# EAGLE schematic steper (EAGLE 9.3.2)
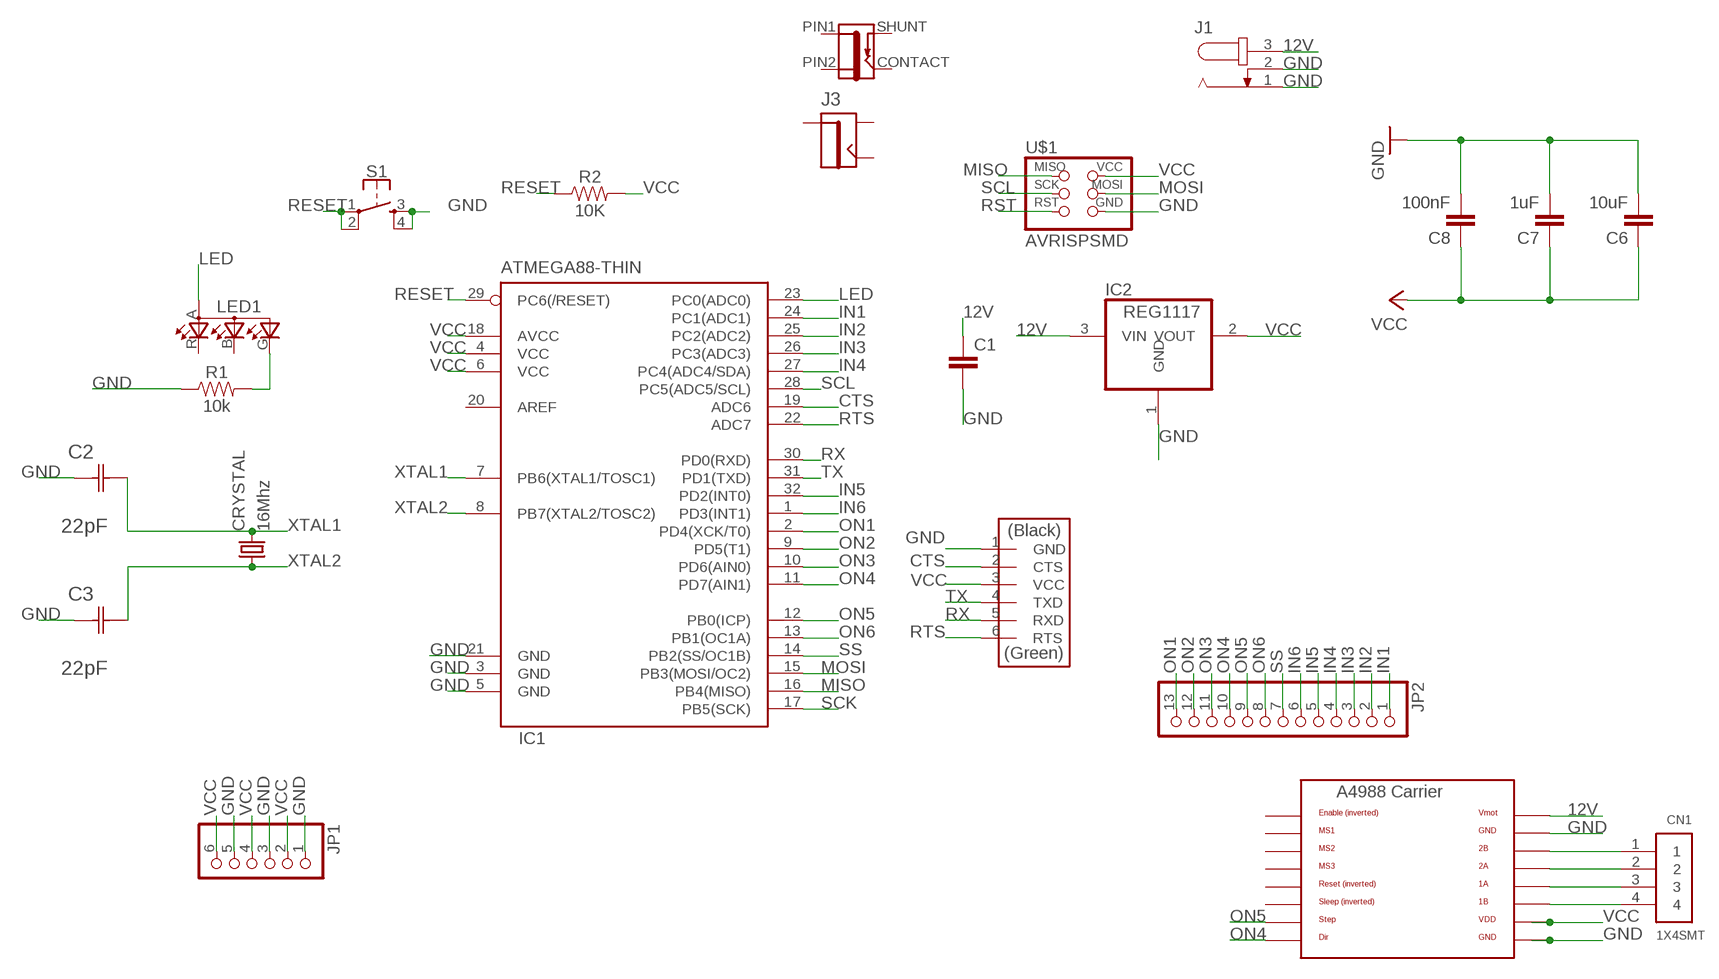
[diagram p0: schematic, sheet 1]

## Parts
C1  C2.5/2  [C2.5-2]
C2  22pF  0612ZC225MAT2A  [CAPC3216X178N]
C3  22pF  0612ZC225MAT2A  [CAPC3216X178N]
C6  10uF  CAP1206  [1206]
C7  1uF  CAP1206  [1206]
C8  100nF  CAP1206  [1206]
CN1  1X4SMT  [1X4-SMT]
CRYSTAL  16Mhz  CSM-7X-DU  [CSM-7X-DU]
IC1  ATMEGA88-THIN  [TQFP32-08THIN]
IC2  REG1117  [SOT223]
J1  JACK-PLUG1  [SPC4078]
J2  JACK-2.1MM  [PJ-002AH-SMT]
J3  JACK2.1MM  [JACK_2.1MM]
JP1  PINHD-1X61X06_SMT  [1X06_SMT]
JP2  PINHD-1X131X13_SMT  [1X13_SMT]
LED1  LEDRGBOLD  [P-LCC-4-3]
R1  10k  10KOHM-0603-1/10W-1%  [0603]
R2  10K  1OHM-0603-1/10W-1%  [0603]
S1  MOMENTARY-SWITCH-SPST-2-SMD-4.6X2.8MM  [TACTILE_SWITCH_SMD_4.6X2.8MM]
U$1  AVRISPSMD  [2X03SMD]
U$2  FTDI-SMD-HEADER  [1X06SMD]
U$4  A4988BREAKOUT  [A4988BREAKOUT]

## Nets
12V: C1.1 IC2.3(VIN) J1.3 U$4.VMOT
CTS: IC1.19(ADC6) U$2.2(CTS)
GND: C1.2 C2.1(C1) C3.1(C1) C6.2 C7.2 C8.2 IC1.3(GND) IC1.5(GND) IC1.21(GND) IC2.1(GND) J1.1 J1.2 JP1.1 JP1.3 JP1.5 R1.1 S1.3 S1.4 U$1.6(GND) U$2.1(GND) U$4.GND U$4.GND@0(GND)
IN1: IC1.24(PC1(ADC1)) JP2.1
IN2: IC1.25(PC2(ADC2)) JP2.2
IN3: IC1.26(PC3(ADC3)) JP2.3
IN4: IC1.27(PC4(ADC4/SDA)) JP2.4
IN5: IC1.32(PD2(INT0)) JP2.5
IN6: IC1.1(PD3(INT1)) JP2.6
LED: IC1.23(PC0(ADC0)) LED1.A(A2)
MISO: IC1.16(PB4(MISO)) U$1.1(MISO)
MOSI: IC1.15(PB3(MOSI/OC2)) U$1.4(MOSI)
N$1: U$4.STEP
N$2: U$4.DIR
N$3: CN1.1 U$4.2B
N$4: CN1.2 U$4.2A
N$5: CN1.3 U$4.1A
N$6: CN1.4 U$4.1B
N$18: LED1.G(CGREEN) R1.2
ON1: IC1.2(PD4(XCK/T0)) JP2.13
ON2: IC1.9(PD5(T1)) JP2.12
ON3: IC1.10(PD6(AIN0)) JP2.11
ON4: IC1.11(PD7(AIN1)) JP2.10
ON5: IC1.12(PB0(ICP)) JP2.9
ON6: IC1.13(PB1(OC1A)) JP2.8
RESET: IC1.29(PC6(/RESET)) R2.1 S1.1 S1.2
RST: U$1.5(RST)
RTS: IC1.22(ADC7) U$2.6(RTS)
RX: IC1.30(PD0(RXD)) U$2.5(RXD)
SCK: IC1.17(PB5(SCK))
SCL: IC1.28(PC5(ADC5/SCL)) U$1.3(SCK)
SS: IC1.14(PB2(SS/OC1B)) JP2.7
TX: IC1.31(PD1(TXD)) U$2.4(TXD)
VCC: C6.1 C7.1 C8.1 IC1.4(VCC) IC1.6(VCC) IC1.18(AVCC) IC2.2(VOUT) JP1.2 JP1.4 JP1.6 R2.2 U$1.2(VCC) U$2.3(VCC) U$4.VDD
XTAL1: C2.2(C2) CRYSTAL.2 IC1.7(PB6(XTAL1/TOSC1))
XTAL2: C3.2(C2) CRYSTAL.1 IC1.8(PB7(XTAL2/TOSC2))
Unconnected: IC1.20(AREF) J3.CONTACT J3.PIN J3.SHUNT LED1.B(CBLUE) LED1.R(CRED) U$4.EN U$4.MS1 U$4.MS2 U$4.MS3 U$4.RST U$4.SLP(SLEEP)

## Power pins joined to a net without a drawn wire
CONTACT: J2.CONTACT
PIN1: J2.PIN1
PIN2: J2.PIN2
SHUNT: J2.SHUNT

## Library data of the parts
C1 = capacitor-wima:C: CAPACITOR
C2 C3 = AVX_By_element14_Batch_1:0612ZC225MAT2A: Capacitor 1206; MPN: 0612ZC225MAT2A; OC_FARNELL: -; OC_NEWARK: 12N3209; SUPPLIER: AVX; TOLERANCE: ±20%; VALUE: 2.2µF; VOLTAGERATING: 10V
C6-C8 = 01_SparkFun:CAP: Capacitor
CN1 = adafruit:1X4: 4-pin connector
CRYSTAL = 01_FAB_Hello:CSM-7X-DU: SMD CRYSTAL; OC_FARNELL: unknown; OC_NEWARK: unknown
IC1 = fab:ATMEGA88-THIN
IC2 = burr-brown:REG1117: 800mA and 1A Low Dropout (LDO) Positive Regulator 1.8V, 2.5V, 2.85V, 3.3V, 5V, and Adj; MPN: REG1117; OC_FARNELL: 1097566; OC_NEWARK: 14P6981
J1 = con-jack:JACK-PLUG: DC POWER JACK Power Jack, DC, Right Angle, Through Hole, Rated 5A at 16VDC, PC Terminals Distributor: Farnell (www.Farnell.de) Drawing: 84N1161.pdf / 84N1162.pdf Manufacturer: SPC Technology (www.spctechnology.com) Type: SPC4077 / SPC 4078; OC_FARNELL: unknown; OC_NEWARK: unknown
J2 = fab:JACK-2.1MM: SMD DC power jack PJ-002AH-SMT As found in the fablab inventory. Made by Zaerc.
J3 = fab:JACK
JP1 = smd_con:PINHD-1X6: PIN HEADER
JP2 = smd_con:PINHD-1X13: PIN HEADER
LED1 = fab:LEDRGBOLD: OSRAM Hyper Multi TOPLED® Hyper-Bright LED LATB T686 Source: http://www.osram.convergy.de/
R1 = SparkFun-Resistors:10KOHM: 10kΩ resistor; PROD_ID: RES-00824
R2 = SparkFun-Resistors:1OHM: 1Ω resistor; PROD_ID: RES-08269; VALUE: 1
S1 = SparkFun-Switches:MOMENTARY-SWITCH-SPST-2: Momentary Switch (Pushbutton) - SPST - Two Circuits Normally-open (NO) SPST momentary switches (buttons, pushbuttons). Schematic symbol includes two switch circuits. Variants SMD-4.6MMX2.8MM - 4.60mm x 2.80mm Tactile Momentary Button Switch - Used on SparkFun SAMD21 Mini Breakout SMD-5.2MM - Mini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; PROD_ID: SWCH-13065
U$1 = fab:AVRISP
U$2 = fab:FTDI-SMD-HEADER
U$4 = RepRapjr:A4988BREAKOUT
